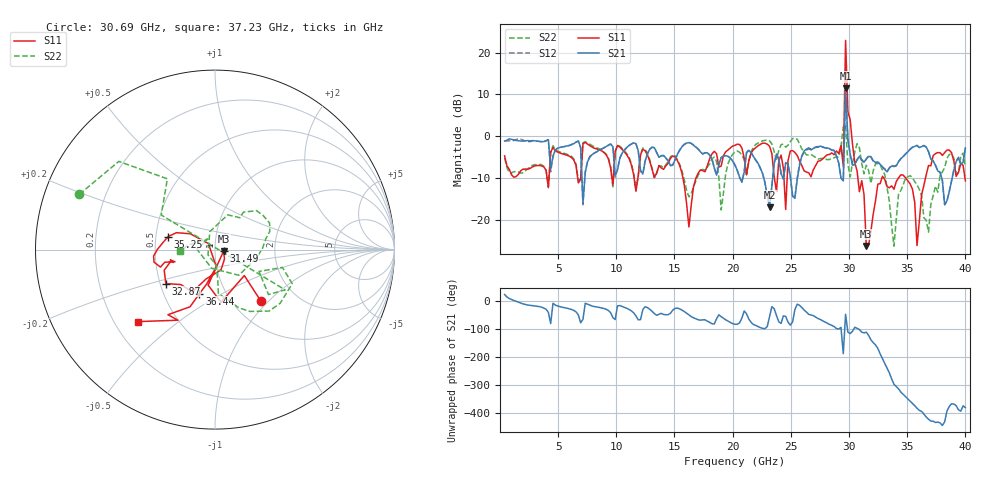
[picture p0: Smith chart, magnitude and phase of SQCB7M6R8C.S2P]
! Network Analyzer HP8722ES.07.66: Jul 25, 2000 Serial No. US39175408
! 26 Oct 2004  15:34:31
! Frequency  S11  S21  S12  S22
# HZ  S  DB R  50
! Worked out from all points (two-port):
!   201 points, 400 MHz to 40 GHz, reference 50 ohm
!   highest |S21| = 11.45 dB at 29.7 GHz (marker M1); lowest = -16.9 dB at 23.17 GHz (marker M2)
!   |S21| within 3 dB of the highest: 29.67707 GHz to 29.75313 GHz (76.06 MHz wide, 0.256 % of centre)
!   lowest |S11| = -26.2 dB at 31.49 GHz (marker M3), VSWR 1.10, Z = 55.1 - j0.88 ohm
!   |S11| at or under -10 dB: 15.73 GHz to 16.84 GHz (1.113 GHz wide, 6.84 % of centre); 30.76 GHz to 32.82 GHz (2.059 GHz wide, 6.48 % of centre); 34.88 GHz to 36.57 GHz (1.688 GHz wide, 4.73 % of centre)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
!   |S22| runs from -26.2 to 2.7 dB; largest |S21 - S12| = 1.6
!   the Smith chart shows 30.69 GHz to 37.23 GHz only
!   S11 on the Smith chart (normalised r, x): 30.69 GHz: 1.34, -0.90; 31.49 GHz: 1.10, -0.02; 32.87 GHz: 0.54, -0.23; 35.25 GHz: 0.58, +0.09; 36.44 GHz: 0.75, -0.40; 37.23 GHz: 0.30, -0.36
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4e8  -4.67 -67.3  -1.13 24.7  -1.11 28.3  -5.23 -60.7
6.736e9  -11.12 -121.2  -1.14 -48.8  -1.08 -49.2  -10.55 -130.8
7.132e9  -1.83 -61.6  -15.98 -64.7  -16.36 -61.5  -1.57 -72.4
1.3666e10  -7.01 -62.8  -5.02 -46.4  -4.97 -45.5  -6.99 -73.6
1.624e10  -21.63 -49.6  -1.50 -48.2  -1.49 -48.1  -14.46 -60.8
2.02e10  -2.16 -12.4  -6.95 -82.2  -6.82 -81.8  -3.72 -2.4
2.317e10  -2.39 -53.6  -16.92 -54.4  -16.93 -51.0  -1.09 -18.6
2.4556e10  -17.46 -2.0  -6.37 -53.6  -6.30 -53.5  -2.60 -6.4
2.6932e10  -7.99 76.5  -2.90 -51.1  -2.71 -52.7  -4.70 -10.0
2.9506e10  -7.13 -2.3  -10.61 172.2  -10.61 -147.1  2.28 27.1
2.9704e10  22.89 3.4  11.45 -46.3  10.39 -21.5  2.72 -65.7
2.9902e10  5.90 -151.9  -0.64 -110.5  -0.80 -109.8  -6.68 -25.1
3.0496e10  -6.32 160.1  -6.74 -92.9  -6.83 -91.3  -3.68 -3.1
3.0694e10  -8.30 -48.3  -5.55 -96.8  -5.61 -95.5  -1.76 157.8
3.1486e10  -26.21 -9.4  -5.41 -110.6  -5.40 -111.4  -6.92 -29.9
3.2872e10  -9.54 -145.4  -7.31 154.3  -7.35 153.0  -8.07 -60.7
3.3466e10  -12.28 -162.8  -7.60 103.2  -7.52 103.2  -15.58 -84.7
3.5248e10  -11.35 164.4  -3.11 2.0  -3.04 1.7  -9.41 25.9
3.5842e10  -26.09 137.5  -2.22 -23.7  -2.16 -23.6  -11.58 0.9
3.6436e10  -11.68 -109.5  -2.23 -44.7  -2.18 -44.5  -19.49 -100.1
3.7228e10  -4.63 -136.9  -5.86 -70.3  -5.84 -69.4  -14.20 -177.2
4e10  -10.64 -167.2  -2.80 -21.6  -2.73 -20.6  -7.15 117.9
